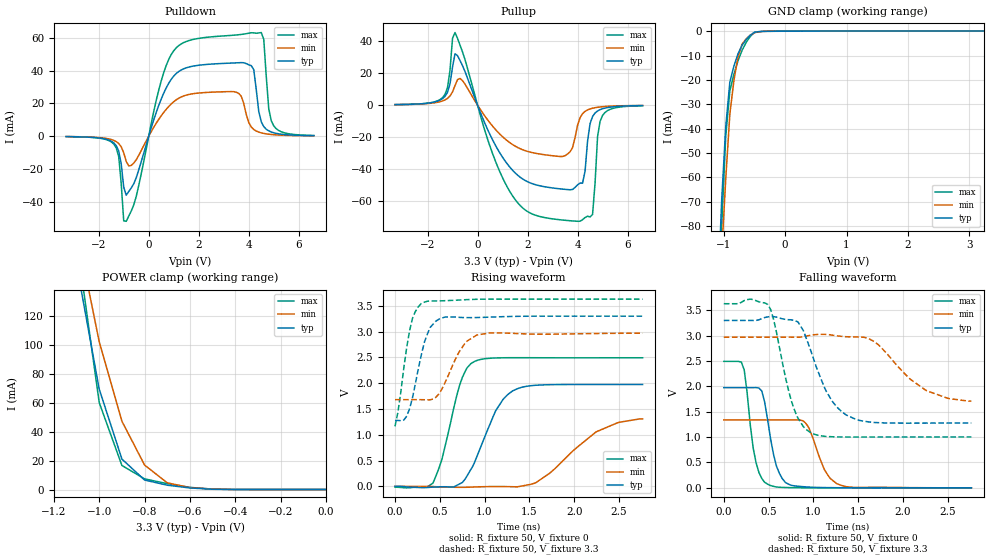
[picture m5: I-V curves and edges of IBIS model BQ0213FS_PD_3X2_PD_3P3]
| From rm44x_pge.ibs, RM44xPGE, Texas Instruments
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|   Model Cell BQ0213FS_PD_3X2_PD_3P3
|BQ0213FS_PD_3X2_PD_3P3
[Model]   BQ0213FS_PD_3X2_PD_3P3
Model_type   I/O
Polarity   Non-Inverting
Enable   Active-Low
Vinl =  1.25
Vinh =  1.65
Cref =  15.0001pF
Rref =  101.0000M
Vref =  0V
Vmeas =  1.65
C_comp   1.2p   1.2p   1.2p
[Model Spec]
Vinl   1.25   1.12   1.38
Vinh   1.65   1.45   1.75
[Temperature Range]   25   155   -40
[Voltage Range]   3.3   2.97   3.63
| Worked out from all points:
|   slope of the pulldown table from 0 to 0.495 V, typ, clamps not added: 22 ohm
|   slope of the pullup table from 0 to 0.495 V, typ, clamps not added: 26.9 ohm
|   GND clamp passes 1 mA (typ) near -0.53 V on its own axis
|   POWER clamp passes 1 mA (typ) near -0.58 V on its own axis
|   rising waveform, R_fixture 50, V_fixture 0: 20-80 % time 297ps typ, 507ps min, 211ps max; typ from 0 V to 1.97 V
|   rising waveform, R_fixture 50, V_fixture 3.3: 20-80 % time 160ps typ, 219ps min, 128ps max; typ from 1.28 V to 3.3 V
|   falling waveform, R_fixture 50, V_fixture 0: 20-80 % time 129ps typ, 181ps min, 108ps max; typ from 1.97 V to 0.001 V
|   falling waveform, R_fixture 50, V_fixture 3.3: 20-80 % time 290ps typ, 442ps min, 208ps max; typ from 3.3 V to 1.28 V
[POWER_clamp]
|   voltage   I(typ)   I(min)   I(max)
-3.3V     2.375A     2.63A      3.153A
-1.1V     156mA      180.2mA    173.4mA
-1.067V   127.2mA    154.3mA    135.7mA
-1.033V   98.46mA    128.4mA    98.04mA
-1V       69.67mA    102.5mA    60.33mA
-900mV    21.21mA    47.43mA    16.77mA
-800mV    6.67mA     17.03mA    7.475mA
-700mV    3.094mA    4.728mA    4.157mA
-600mV    1.183mA    1.448mA    1.593mA
-500mV    283.5uA    402.1uA    371.9uA
0V        96.5uA     44.21uA    168.6uA
[Pulldown]
|   voltage   I(typ)   I(min)   I(max)
-3.3V     -269.8uA   -248.1uA   -260.2uA
-1.4V     -4.056mA   -2.548mA   -4.78mA
-1.2V     -9.105mA   -4.482mA   -12.53mA
-900mV    -36.12mA   -15.43mA   -52.09mA
1V        36.78mA    21.07mA    52.28mA
3.5V      44.86mA    26.92mA    61.93mA
4.1V      43.14mA    5.644mA    63.29mA
4.5V      8.805mA    2.025mA    63.4mA
4.6V      5.861mA    1.678mA    59.29mA
4.8V      3.241mA    1.203mA    16.69mA
5V        2.072mA    900.6uA    6.272mA
6.6V      302.2uA    232.4uA    414.2uA
[Pullup]
|   voltage   I(typ)   I(min)   I(max)
-3.3V     296.7uA    284.3uA    270.4uA
-1.4V     3.997mA    2.582mA    4.655mA
-1.2V     8.017mA    4.201mA    10.97mA
-900mV    32.15mA    12.24mA    45.44mA
1.4V      -40.82mA   -24.72mA   -56.86mA
3.4V      -52.65mA   -32.22mA   -72.03mA
4V        -49.98mA   -12.64mA   -72.82mA
4.2V      -48.91mA   -5.386mA   -71.82mA
4.6V      -7.16mA    -1.965mA   -68.53mA
4.8V      -3.684mA   -1.373mA   -19.8mA
5V        -2.282mA   -1.01mA    -6.487mA
6.6V      -316.6uA   -254.8uA   -401.1uA
[GND_clamp]
|   voltage   I(typ)   I(min)   I(max)
-3.3V     -1.947A    -1.623A    -3.254A
-1.1V     -112mA     -127.1mA   -135.8mA
-1.033V   -69.62mA   -91.64mA   -80.2mA
-966.7mV  -39.25mA   -60.63mA   -43.13mA
-900mV    -20.89mA   -34.03mA   -24.55mA
-833.3mV  -14.3mA    -20.13mA   -17.67mA
-766.7mV  -9.242mA   -10.53mA   -12.09mA
-700mV    -5.726mA   -5.229mA   -7.796mA
-566.7mV  -1.616mA   -1.599mA   -2.13mA
-500mV    -447.1uA   -610uA     -527.1uA
-300mV    -27.38uA   -21.6uA    -40.6uA
3.233V    96.49uA    48.22uA    168.5uA
[Ramp]
| variable   typ   min   max
dV/dt_f   1.261182/0.2949071n  0.8128074/0.4784683n   1.630758/0.2132796n
dV/dt_r   1.199734/0.3017159n  0.8149211/0.5359589n   1.513262/0.2083871n
R_load = 50
[Rising Waveform]
R_fixture = 50
V_fixture = 0
V_fixture_min = 0
V_fixture_max = 0
|   time   V(typ)   V(min)   V(max)
0s        -29.58uV   10.33uV    -14.58mV
424ps     -14.14mV   -3.238mV   63.49mV
524ps     -7.805mV   -11.93mV   523.6mV
720ps     46.93mV    -17.93mV   1.952V
888ps     463.9mV    -11.26mV   2.421V
1.124ns   1.466V     -3.033mV   2.488V
1.312ns   1.849V     -6.711mV   2.493V
1.568ns   1.959V     66.47mV    2.492V
2.24ns    1.974V     1.049V     2.491V
2.764ns   1.974V     1.307V     2.492V
[Rising Waveform]
R_fixture = 50
V_fixture = 3.3
V_fixture_min = 2.97
V_fixture_max = 3.63
|   time   V(typ)   V(min)   V(max)
0s        1.278V     1.68V      1.163V
100ps     1.289V     1.68V      2.316V
164ps     1.511V     1.68V      3.026V
228ps     1.992V     1.68V      3.39V
296ps     2.564V     1.679V     3.548V
392ps     3.077V     1.677V     3.592V
456ps     3.202V     1.726V     3.593V
720ps     3.275V     2.617V     3.611V
912ps     3.271V     2.931V     3.625V
2.764ns   3.298V     2.968V     3.628V
[Falling Waveform]
R_fixture = 50
V_fixture = 0
V_fixture_min = 0
V_fixture_max = 0
|   time   V(typ)   V(min)   V(max)
0s        1.974V     1.338V     2.492V
228ps     1.974V     1.338V     2.324V
360ps     1.976V     1.338V     497mV
492ps     1.311V     1.338V     69.99mV
588ps     429.1mV    1.338V     17.02mV
752ps     50.98mV    1.338V     4.519mV
912ps     19.4mV     1.279V     1.158mV
1.124ns   5.651mV    356.9mV    635.5uV
1.312ns   2.243mV    48.49mV    832uV
2.764ns   534.4uV    530.5uV    42.77uV
[Falling Waveform]
R_fixture = 50
V_fixture = 3.3
V_fixture_min = 2.97
V_fixture_max = 3.63
|   time   V(typ)   V(min)   V(max)
0s        3.298V     2.969V     3.628V
492ps     3.369V     2.969V     3.613V
752ps     3.311V     2.969V     1.725V
828ps     3.271V     2.968V     1.372V
976ps     2.679V     3.009V     1.078V
1.208ns   1.711V     3.01V      1.007V
1.464ns   1.359V     2.974V     1.001V
1.724ns   1.284V     2.822V     1.002V
2.264ns   1.276V     1.914V     1.003V
2.764ns   1.278V     1.709V     1.003V
